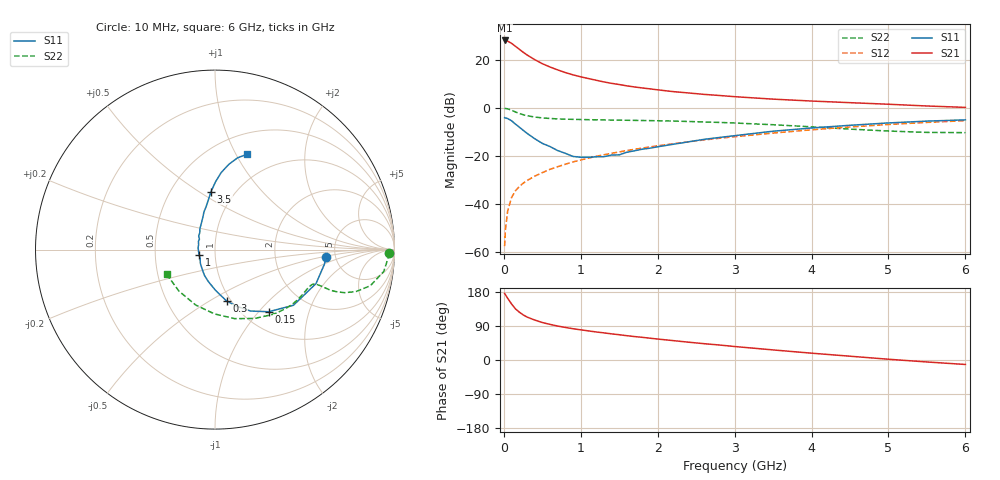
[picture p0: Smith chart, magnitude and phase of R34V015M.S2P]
! SIEMENS Small Signal Semiconductors
! BFR181
! Si NPN RF Bipolar Junction Transistor in SOT23
! VCE = 4 V  IC = 15 mA
! Common Emitter S-Parameters:  May  1996
# GHz  S  MA  R  50
!  f  S11  S21  S12  S22
! GHz  MAG  ANG  MAG  ANG  MAG  ANG  MAG  ANG
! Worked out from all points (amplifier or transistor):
!   36 points, 10 MHz to 6 GHz, reference 50 ohm
!   highest |S21| = 28.1 dB at 10 MHz (marker M1)
!   |S21| within 3 dB of that: start of sweep to 173.8 MHz
!   unconditionally stable (mu >= 1): 617.5 MHz to 2.547 GHz
!   at 250 MHz: K = 0.72, MSG = 27.3 dB, |S12| = -31.5 dB
!   at 1.4 GHz: K = 1.07, MAG = 12.9 dB, |S12| = -19.0 dB
!   at 6 GHz: K = 0.86, MSG = 2.8 dB, |S12| = -5.4 dB
!   S11 on the Smith chart (normalised r, x): 10 MHz: 4.21, -0.57; 150 MHz: 1.29, -1.13; 300 MHz: 0.96, -0.60; 1 GHz: 0.84, -0.05; 3.5 GHz: 0.78, +0.56; 6 GHz: 0.72, +1.11
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0.01  0.6217 -3.8  25.29 175.9  0.0013 86.2  0.9722 -1.2
0.02  0.6148 -7.7  25.12 172.5  0.0028 84.0  0.9649 -3.0
0.05  0.5938 -18.6  24.48 162.7  0.0071 81.1  0.9481 -7.4
0.1  0.5357 -35.4  22.01 148.0  0.0134 76.3  0.8886 -13.1
0.15  0.4572 -49.2  19.16 135.1  0.0185 71.2  0.819 -16.6
0.2  0.3957 -59.9  16.62 126.4  0.0227 71.6  0.7608 -18.4
0.25  0.3403 -68.6  14.44 119.2  0.0266 69.2  0.7174 -19.1
0.3  0.2943 -77.2  12.66 113.5  0.0302 70.3  0.6838 -19.4
0.4  0.2269 -89.3  10.1 105.5  0.0374 71.2  0.6408 -19.1
0.5  0.1807 -102.2  8.298 98.9  0.0443 71.5  0.6138 -18.9
0.6  0.1552 -112.3  7.074 94.0  0.052 72.0  0.5977 -18.9
0.7  0.128 -124.5  6.153 89.6  0.059 72.8  0.5856 -19.2
0.8  0.112 -136.8  5.413 85.9  0.0664 72.8  0.5782 -19.5
1  0.0928 -162.5  4.416 79.6  0.0815 72.8  0.5683 -20.8
1.1  0.0925 -175.2  4.06 76.8  0.089 72.8  0.5639 -21.6
1.3  0.0952 163.8  3.457 71.6  0.1046 72.0  0.5568 -23.5
1.6  0.1182 140.1  2.858 64.1  0.128 70.8  0.5485 -27.0
2.2  0.1729 115.1  2.171 51.2  0.1778 67.3  0.5274 -35.3
3.5  0.3241 93.9  1.512 26.6  0.2967 56.2  0.4425 -60.1
4.5  0.4308 85.4  1.276 10.0  0.3974 44.8  0.3585 -90.4
5.5  0.5264 76.2  1.088 -5.2  0.4947 31.4  0.3063 -131.0
6  0.5592 71.6  1.017 -11.8  0.5376 24.2  0.3026 -153.1
